FUNCTION "PALLET IMP.POST TRANSITO" : VOID
TITLE =
VERSION : 0.1
//KNOW_HOW_PROTECT

VAR_TEMP
  Error_block_move : INT ;
END_VAR
BEGIN
NETWORK
TITLE =Spostamento dati per pallet in transito tra impil. e ribaltat.
//- "Container Flag"
//- "Id TAG"
//- "FlagRibaltamento"
//- "Container_Id"
//- "Date LCB"
//- "Part Number"
//- "Quantity"
//- "Line Id"
//- "CIM"
//- "Colata Id"
//- "Material Of Test Flag"
//- "Lotto Id"
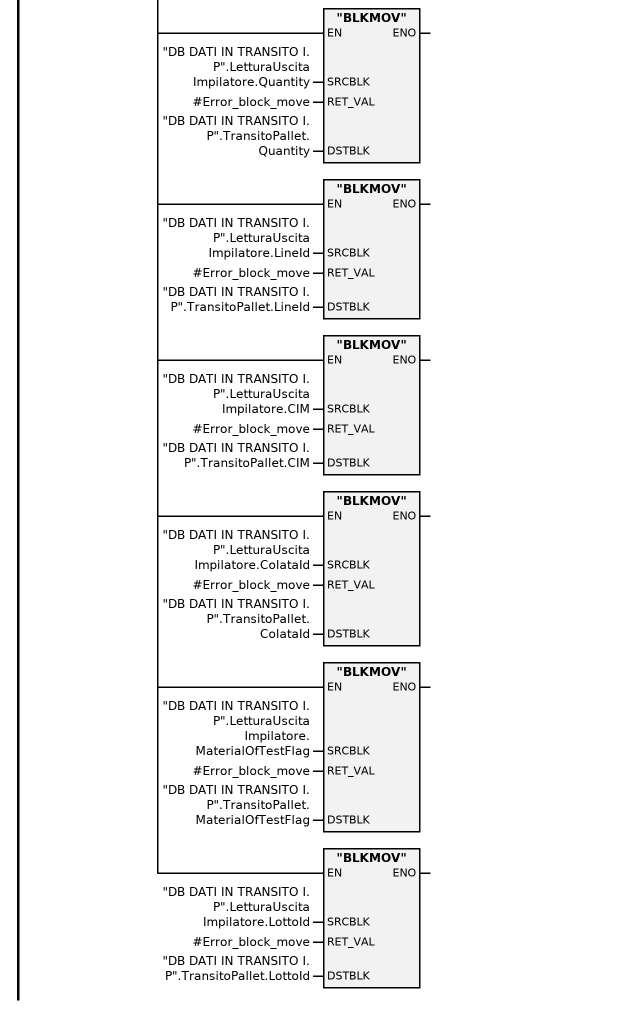
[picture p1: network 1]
      U     "DB SCAMBIO DATI PIANELLI".Trasl_ped_da_I_P_a_ribal;
      =     L      2.0;
      U     L      2.0;
      SPBNB _001;
      CALL "BLKMOV" (
           SRCBLK                   := "DB DATI IN TRANSITO I. P".LetturaUscitaImpilatore.ContainerFlag,
           RET_VAL                  := #Error_block_move,
           DSTBLK                   := "DB DATI IN TRANSITO I. P".TransitoPallet.ContainerFlag);
_001: NOP   0;
      U     L      2.0;
      SPBNB _002;
      CALL "BLKMOV" (
           SRCBLK                   := "DB DATI IN TRANSITO I. P".LetturaUscitaImpilatore.ID_TAG,
           RET_VAL                  := #Error_block_move,
           DSTBLK                   := "DB DATI IN TRANSITO I. P".TransitoPallet.ID_TAG);
_002: NOP   0;
      U     L      2.0;
      SPBNB _003;
      CALL "BLKMOV" (
           SRCBLK                   := "DB DATI IN TRANSITO I. P".LetturaUscitaImpilatore.FlagRibaltamento,
           RET_VAL                  := #Error_block_move,
           DSTBLK                   := "DB DATI IN TRANSITO I. P".TransitoPallet.FlagRibaltamento);
_003: NOP   0;
      U     L      2.0;
      SPBNB _004;
      CALL "BLKMOV" (
           SRCBLK                   := "DB DATI IN TRANSITO I. P".LetturaUscitaImpilatore.Container_Id,
           RET_VAL                  := #Error_block_move,
           DSTBLK                   := "DB DATI IN TRANSITO I. P".TransitoPallet.Container_Id);
_004: NOP   0;
      U     L      2.0;
      SPBNB _005;
      CALL "BLKMOV" (
           SRCBLK                   := "DB DATI IN TRANSITO I. P".LetturaUscitaImpilatore.DateLCB,
           RET_VAL                  := #Error_block_move,
           DSTBLK                   := "DB DATI IN TRANSITO I. P".TransitoPallet.DateLCB);
_005: NOP   0;
      U     L      2.0;
      SPBNB _006;
      CALL "BLKMOV" (
           SRCBLK                   := "DB DATI IN TRANSITO I. P".LetturaUscitaImpilatore.PartNumber,
           RET_VAL                  := #Error_block_move,
           DSTBLK                   := "DB DATI IN TRANSITO I. P".TransitoPallet.PartNumber);
_006: NOP   0;
      U     L      2.0;
      SPBNB _007;
      CALL "BLKMOV" (
           SRCBLK                   := "DB DATI IN TRANSITO I. P".LetturaUscitaImpilatore.Quantity,
           RET_VAL                  := #Error_block_move,
           DSTBLK                   := "DB DATI IN TRANSITO I. P".TransitoPallet.Quantity);
_007: NOP   0;
      U     L      2.0;
      SPBNB _008;
      CALL "BLKMOV" (
           SRCBLK                   := "DB DATI IN TRANSITO I. P".LetturaUscitaImpilatore.LineId,
           RET_VAL                  := #Error_block_move,
           DSTBLK                   := "DB DATI IN TRANSITO I. P".TransitoPallet.LineId);
_008: NOP   0;
      U     L      2.0;
      SPBNB _009;
      CALL "BLKMOV" (
           SRCBLK                   := "DB DATI IN TRANSITO I. P".LetturaUscitaImpilatore.CIM,
           RET_VAL                  := #Error_block_move,
           DSTBLK                   := "DB DATI IN TRANSITO I. P".TransitoPallet.CIM);
_009: NOP   0;
      U     L      2.0;
      SPBNB _00a;
      CALL "BLKMOV" (
           SRCBLK                   := "DB DATI IN TRANSITO I. P".LetturaUscitaImpilatore.ColataId,
           RET_VAL                  := #Error_block_move,
           DSTBLK                   := "DB DATI IN TRANSITO I. P".TransitoPallet.ColataId);
_00a: NOP   0;
      U     L      2.0;
      SPBNB _00b;
      CALL "BLKMOV" (
           SRCBLK                   := "DB DATI IN TRANSITO I. P".LetturaUscitaImpilatore.MaterialOfTestFlag,
           RET_VAL                  := #Error_block_move,
           DSTBLK                   := "DB DATI IN TRANSITO I. P".TransitoPallet.MaterialOfTestFlag);
_00b: NOP   0;
      U     L      2.0;
      SPBNB _00c;
      CALL "BLKMOV" (
           SRCBLK                   := "DB DATI IN TRANSITO I. P".LetturaUscitaImpilatore.LottoId,
           RET_VAL                  := #Error_block_move,
           DSTBLK                   := "DB DATI IN TRANSITO I. P".TransitoPallet.LottoId);
_00c: NOP   0;
NETWORK
TITLE =
//m20000.0 = Tag corrispondente
//
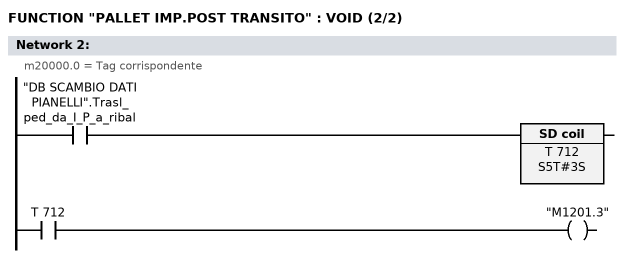
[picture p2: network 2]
      U     "DB SCAMBIO DATI PIANELLI".Trasl_ped_da_I_P_a_ribal;
      L     S5T#3S;
      SE    T    712;
      NOP   0;
      NOP   0;
      NOP   0;
      U     T    712;
      =     "M1201.3";
END_FUNCTION

